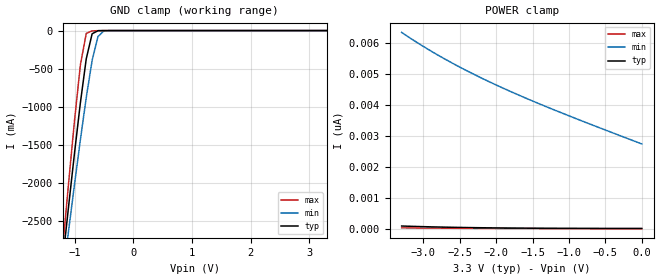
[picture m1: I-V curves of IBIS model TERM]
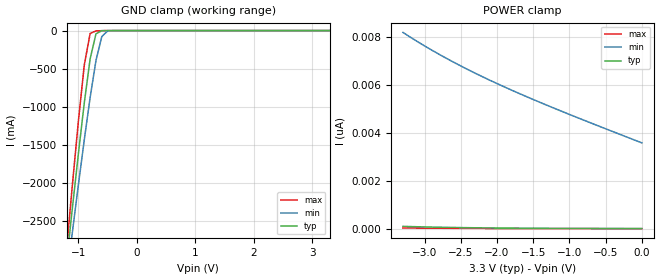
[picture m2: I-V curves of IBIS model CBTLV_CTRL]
| I/O Buffer Information Specification (IBIS) Version 3.2 (August 20, 1999)
| IBIS is a standard for electronic behavioral specifications of integrated
| circuit input/output analog characteristics.
[IBIS Ver]   3.2
[File Name]   cbtlv16210.ibs
[File Rev]   1.1
[Date]   Wednesday, September 4, 2002
[Source]   Integrated Device Technology, Inc.
[Notes]   1.Temperatures: typ=25C, min=-40C, max=100C
[Disclaimer] Integrated Device Technology, Inc. ("IDT") hereby grants the
   user of this IBIS model a non-exclusive, nontransferable
   license to use this IBIS model under the following terms. The
   user is granted this license only to use the IBIS model and is
   not granted rights to sell, copy (except as needed to run the
   IBIS model), rent, lease or sub-license the IBIS model in
   whole or in part, or in modified form to anyone. The User may
   modify the IBIS model to suit its specific applications, but
   rights to derivative works and such modifications shall belong
   to IDT.
   This IBIS model is provided on an "AS IS" basis and IDT
   makes absolutely no warranty with respect to the information
   contained herein. IDT DISCLAIMS AND CUSTOMER WAIVES ALL
   WARRANTIES, EXPRESS AND IMPLIED, INCLUDING WARRANTIES OF
   MERCHANTABILITY AND FITNESS FOR A PARTICULAR PURPOSE. THE
   ENTIRE RISK AS TO QUALITY AND PERFORMANCE IS WITH THE USER
   ACCORDINGLY, IN NO EVENT SHALL IDT BE LIABLE FOR ANY DIRECT OR
   INDIRECT DAMAGES, WHETHER IN CONTRACT OR TORT,  INCLUDING
   ANY LOST PROFITS OR OTHER INCIDENTAL, CONSEQUENTIAL, EXEMPLARY
   OR PUNITIVE DAMAGES ARISING OUT OF THE USE OR APPLICATION OF
   THE IBIS model.
   Further, IDT reserves the right to make changes without notice
   to any product herein to improve reliability, function, or
   design. IDT does not convey any license under patent rights or
   any other intellectual property rights, including those of
   third parties. IDT is not obligated to provide maintenance or
   support for the licensed IBIS model.
[Copyright]   Copyright 1997, Integrated Device Technology, Inc. all rights
   reserved.
|   Component IDT74CBTLV16210
[Component]   IDT74CBTLV16210
[Manufacturer]   Integrated Device Technology
[Package]
|Following package parameters are for 48 lead Shrink Small Outline package
| variable   typ   min   max
R_pkg   6.35000m   5.00000m   10.00000m
L_pkg   5.13000nH   4.49000nH   6.33000nH
C_pkg   0.14300pF   0.07300pF   0.26900pF
[Pin]  signal_name   model_name   R_pin   L_pin   C_pin
1   NC   NC
2   1A1   TERM
3   1A2   TERM
4   1A3   TERM
5   1A4   TERM
6   1A5   TERM
7   1A6   TERM
8   GND   GND
9   1A7   TERM
10   1A8   TERM
11   1A9   TERM
12   1A10   TERM
13   2A1   TERM
14   2A2   TERM
15   VCC   POWER
16   2A3   TERM
17   GND   GND
18   2A4   TERM
19   2A5   TERM
20   2A6   TERM
21   2A7   TERM
22   2A8   TERM
23   2A9   TERM
24   2A10   TERM
25   2B10   TERM
26   2B9   TERM
27   2B8   TERM
28   2B7   TERM
29   2B6   TERM
30   2B5   TERM
31   2B4   TERM
32   GND   GND
33   2B3   TERM
34   2B2   TERM
35   2B1   TERM
36   1B10   TERM
37   1B9   TERM
38   1B8   TERM
39   1B7   TERM
40   1B6   TERM
41   GND   GND
42   1B5   TERM
43   1B4   TERM
44   1B3   TERM
45   1B2   TERM
46   1B1   TERM
47   _2OE_   CBTLV_CTRL
48   _1OE_   CBTLV_CTRL
[Series Switch Groups]
|Function Group States
On A /
On B /
On A B /
Off A B /
[Series Pin Mapping]   pin_2   model_name   function_table_group
2   46   CBTLV_SW   A
3   45   CBTLV_SW   A
4   44   CBTLV_SW   A
5   43   CBTLV_SW   A
6   42   CBTLV_SW   A
7   40   CBTLV_SW   A
9   39   CBTLV_SW   A
10   38   CBTLV_SW   A
11   37   CBTLV_SW   A
12   36   CBTLV_SW   A
13   35   CBTLV_SW   B
14   34   CBTLV_SW   B
16   33   CBTLV_SW   B
18   31   CBTLV_SW   B
19   30   CBTLV_SW   B
20   29   CBTLV_SW   B
21   28   CBTLV_SW   B
22   27   CBTLV_SW   B
23   26   CBTLV_SW   B
24   25   CBTLV_SW   B
|   Model CBTLV_SW
[Model]   CBTLV_SW
Model_type   Series_switch
C_comp   0.00000pF   0.000000pF   0.00000pF
[Temperature Range]   25.00000   100.00000   -40.00000
[Voltage Range]   3.30000V   3.00000V   3.60000V
[On]
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[Off]
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| Models and submodels in the file (3): TERM (Terminator), CBTLV_CTRL (Input), CBTLV_SW (Series_switch)
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|   Model TERM
[Model]   TERM
Model_type   Terminator
C_comp   7.00000pF   7.00000pF   7.00000pF
[Temperature Range]   25.00000   100.00000   -40.00000
[Voltage Range]   3.30000V   3.00000V   3.60000V
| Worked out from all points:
|   GND clamp passes 1 mA (typ) near -0.56 V on its own axis
[GND_clamp]
| voltage   I(typ)   I(min)   I(max)
-3.3V     -18.68A    -16.69A    -21.55A
-1.2V     -3.01A     -3.233A    -2.838A
-1.1V     -2.3A      -2.62A     -1.994A
-1V       -1.607A    -2.018A    -1.181A
-900mV    -948.2mA   -1.433A    -450.8mA
-800mV    -370.4mA   -879mA     -37.74mA
-700mV    -42.23mA   -392.2mA   -4.26mA
-600mV    -1.698mA   -77.63mA   -1.062mA
-500mV    -121.2uA   -4.933mA   -126.2uA
3.3V      6.967pA    3.013nA    1.211pA
[POWER_clamp]
| voltage   I(typ)   I(min)   I(max)
-3.3V     86.64pA    6.353nA    27.63pA
-3V       66.02pA    5.896nA    21.07pA
-2.7V     49.77pA    5.483nA    15.87pA
-2.4V     37.26pA    5.106nA    11.8pA
-2V       25.27pA    4.65nA     7.816pA
-1.6V     17.41pA    4.232nA    5.123pA
-1.2V     12.49pA    3.841nA    3.396pA
0V        6.967pA    2.744nA    1.371pA
|   Model CBTLV_CTRL
[Model]   CBTLV_CTRL
Model_type   Input
Vinl =  0.80000V
Vinh =  2.00000V
C_comp   4.00000pF   4.00000pF   4.00000pF
[Temperature Range]   25.00000   100.00000   -40.00000
[Voltage Range]   3.30000V   3.00000V   3.60000V
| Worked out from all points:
|   GND clamp passes 1 mA (typ) near -0.55 V on its own axis
[GND_clamp]
| voltage   I(typ)   I(min)   I(max)
-3.3V     -18.68A    -16.7A     -21.56A
-1.2V     -3.012A    -3.235A    -2.839A
-1.1V     -2.301A    -2.621A    -1.994A
-1V       -1.608A    -2.019A    -1.181A
-900mV    -948.8mA   -1.433A    -451.3mA
-800mV    -370.8mA   -879.6mA   -38.09mA
-700mV    -42.47mA   -392.6mA   -4.468mA
-600mV    -1.797mA   -77.91mA   -1.149mA
-500mV    -139.7uA   -5.076mA   -143.8uA
3.3V      7.987pA    3.938nA    1.364pA
[POWER_clamp]
| voltage   I(typ)   I(min)   I(max)
-3.3V     97.02pA    8.199nA    30.43pA
-3V       74.04pA    7.633nA    23.23pA
-2.7V     55.91pA    7.117nA    17.53pA
-2.4V     41.93pA    6.643nA    13.05pA
-2V       28.53pA    6.062nA    8.669pA
-1.6V     19.72pA    5.525nA    5.699pA
-1.2V     14.2pA     5.019nA    3.787pA
0V        7.987pA    3.585nA    1.542pA
